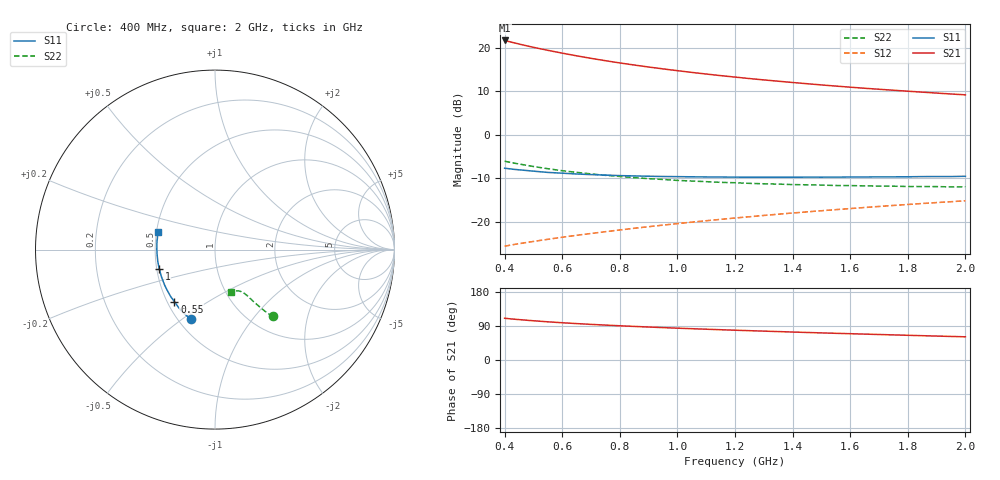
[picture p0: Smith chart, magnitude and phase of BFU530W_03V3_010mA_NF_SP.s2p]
! Filename:  P:\Prog\Test\Noise\ATS_data\Testdata_Net\06 Compressed Noise after Statistics\BFU530W_APM2013_09_A05_03p3V_010mA_NF_CM01_D.sf
! Date/Time: Tue 26/Mar/2013 18:06:07
! BFU530W_APM2013_09_A05_03p3V_1to25mA_NF_CM01_Bias6_R.sf
! Noise Parameter Data File
! BFU530W_APM2013_09_A05_03p3V_1to25mA_NF_CM01
! Date/time: Thu Mar 21 19:18:02 2013
! VAR V_out= 3.300000
! VAR I_out= 9.990000
! VAR V_in= 0.835900
! VAR I_in= 0.108005
! Device data file deembeded for feedlines and parallel
! Original file: \06 Compressed Noise after Statistics\BFU530W_APM2013_09_A05_03p3V_010mA_NF_CM01_R.sf
! Feed-files: PR019V01_070313_Feed1.s2p, PR019V01_070313_Feed2.s2p
! Parallel-file: PR019V01_070313_Par.s2p
# MHz S MA R 50
!  Freq-MHz  S11-mag  S11-arg  S21-mag  S21-arg  S12-mag  S12-arg  S22-mag  S22-arg
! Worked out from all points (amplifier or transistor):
!   37 points, 400 MHz to 2 GHz, reference 50 ohm
!   highest |S21| = 21.6 dB at 400 MHz (marker M1)
!   |S21| within 3 dB of that: start of sweep to 606.9 MHz
!   unconditionally stable (mu >= 1): 1.381 GHz to end of sweep
!   at 500 MHz: K = 0.73, MSG = 22.3 dB, |S12| = -24.6 dB
!   at 1.1 GHz: K = 0.97, MSG = 16.9 dB, |S12| = -19.8 dB
!   at 2 GHz: K = 1.02, MAG = 11.4 dB, |S12| = -15.2 dB
!   lowest NFmin = 0.72 dB at 420 MHz
!   S11 on the Smith chart (normalised r, x): 400 MHz: 0.58, -0.54; 550 MHz: 0.54, -0.37; 1 GHz: 0.52, -0.12; 2 GHz: 0.51, +0.11
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400  0.411 -109.3  12.06 110.1  0.05223 58.9  0.4938 -49.0
420  0.4034 -112.3  11.6 108.6  0.05369 58.9  0.4791 -49.6
433  0.3984 -114.0  11.32 107.8  0.05459 58.9  0.47 -50.0
460  0.3911 -117.6  10.78 106.0  0.05647 59.1  0.4532 -50.6
500  0.3801 -122.6  10.05 103.5  0.0592 59.2  0.4298 -51.3
550  0.3675 -128.0  9.287 100.8  0.0626 59.8  0.4053 -52.0
600  0.3602 -133.1  8.621 98.3  0.06612 60.1  0.3845 -52.7
650  0.3525 -137.6  8.028 96.1  0.0696 60.6  0.3681 -53.1
700  0.3469 -141.8  7.513 94.0  0.07306 61.0  0.3534 -53.7
750  0.3424 -145.5  7.057 92.1  0.07659 61.5  0.3402 -54.0
800  0.3376 -149.2  6.654 90.3  0.08021 61.9  0.3305 -54.5
850  0.3351 -152.5  6.295 88.6  0.0838 62.3  0.32 -54.8
950  0.3299 -158.3  5.684 85.5  0.09115 63.0  0.3049 -55.6
1000  0.3287 -161.2  5.421 84.0  0.09486 63.2  0.2974 -55.8
1100  0.326 -166.1  4.96 81.2  0.1024 63.7  0.2878 -56.9
1200  0.3242 -170.6  4.575 78.6  0.11 64.0  0.2796 -57.8
1250  0.3238 -172.9  4.402 77.4  0.1138 64.1  0.2752 -58.2
1350  0.3235 -176.6  4.102 75.0  0.1216 64.2  0.2698 -59.3
1500  0.3241 177.8  3.719 71.5  0.1334 64.2  0.263 -61.3
1650  0.3255 172.7  3.405 68.3  0.1453 64.1  0.2574 -63.2
1750  0.3268 169.9  3.232 66.2  0.1533 63.9  0.2552 -64.6
2000  0.3318 162.7  2.86 61.2  0.1735 63.1  0.2511 -68.7
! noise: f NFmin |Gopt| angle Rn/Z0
400  0.7631  0.09205  165.5  0.077
460  0.7613  0.09804  165.1  0.0785
600  0.7824  0.1064  169.7  0.0783
800  0.8182  0.1347  170.4  0.0732
1000  0.8374  0.1494  174.7  0.0736
1200  0.8901  0.1698  172.3  0.073
1400  0.9032  0.1936  -178.5  0.0648
1600  0.9166  0.234  -173.6  0.0629
1800  0.9687  0.2382  -171.9  0.063
2000  0.9828  0.2471  -167.1  0.072
